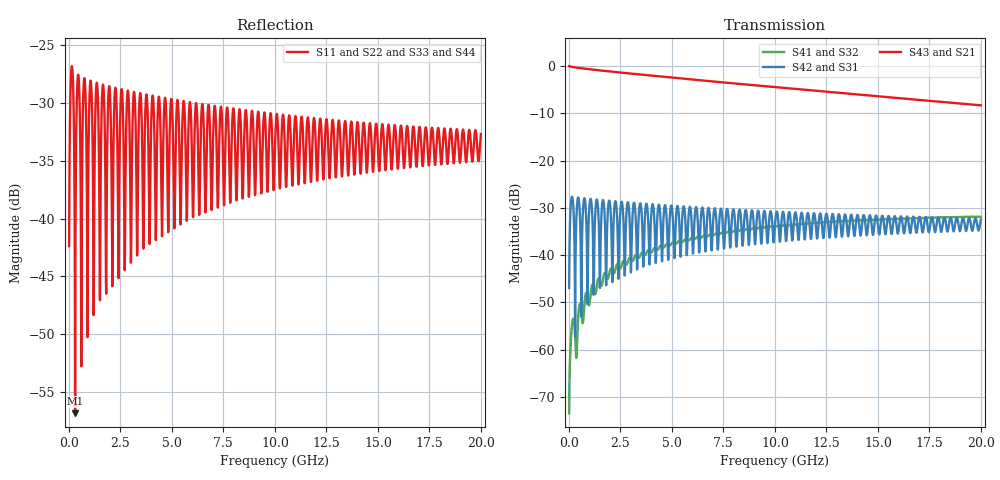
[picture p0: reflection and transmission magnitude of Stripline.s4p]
# Hz S RI R 50
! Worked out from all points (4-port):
!   2000 points, 10 MHz to 20 GHz, reference 50 ohm
!   strongest paths, dB at 10 MHz, 5.01 GHz, 10.01 GHz, 15.01 GHz, 20 GHz:
!     S43: 0.0, -2.5, -4.5, -6.4, -8.3
!     S21: 0.0, -2.5, -4.5, -6.4, -8.3
!     S42: -47.0, -30.2, -33.3, -34.1, -32.5
!     S31: -47.0, -30.2, -33.3, -34.1, -32.5
!     S41: -73.5, -37.4, -34.0, -32.4, -31.9
!     S32: -73.5, -37.4, -34.0, -32.4, -31.9
!   lowest |S11| = -56.8 dB at 300 MHz (marker M1), VSWR 1.00, Z = 50.1 - j0.0299 ohm
!   |S11| at or under -10 dB: start of sweep to end of sweep
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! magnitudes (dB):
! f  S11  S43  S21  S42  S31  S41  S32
! 10 MHz  -42.4  0.0  0.0  -47.0  -47.0  -73.5  -73.5
! 140 MHz  -26.8  -0.2  -0.2  -27.7  -27.7  -55.1  -55.2
! 300 MHz  -56.8  -0.3  -0.3  -57.3  -57.3  -56.6  -56.6
! 450 MHz  -27.6  -0.4  -0.4  -27.8  -27.8  -53.1  -53.1
! 1.44 GHz  -32.2  -0.9  -0.9  -32.2  -32.2  -44.9  -44.9
! 4.75 GHz  -32.8  -2.3  -2.4  -32.7  -32.7  -37.6  -37.6
! 20 GHz  -32.7  -8.3  -8.3  -32.5  -32.5  -31.9  -31.9
